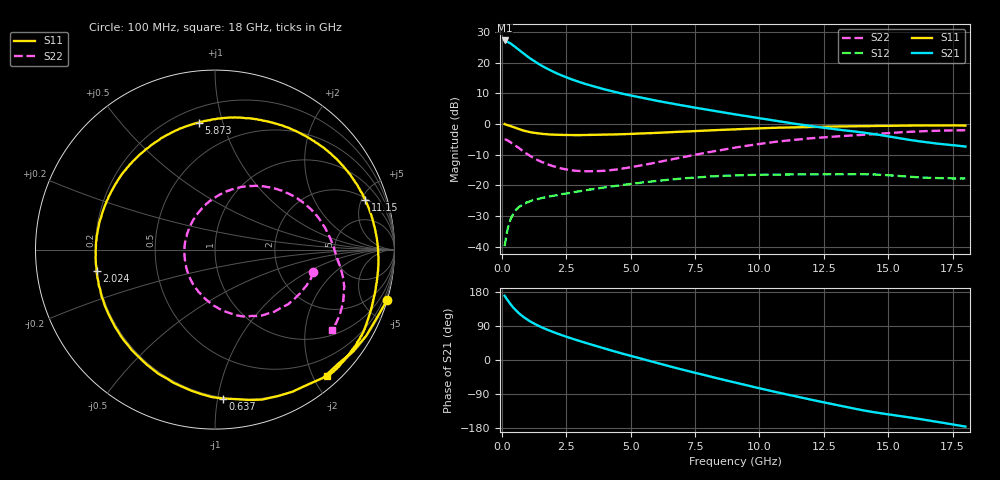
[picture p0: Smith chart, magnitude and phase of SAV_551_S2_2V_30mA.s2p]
! Data provided by Modelithics, Inc.  Tampa, Florida USA, June 2008
!Model SAV-551+
!VAR V_out= 2
!VAR I_out= 30
!VAR V_in= 0.3940
!VAR I_in= 0.9720
!BEGIN ACDATA
# GHZ S MA R 50
! Scattering Parameters
!% F n11x n11y n21x n21y n12x n12y n22x n22y
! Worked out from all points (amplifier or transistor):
!   401 points, 100 MHz to 18 GHz, reference 50 ohm
!   highest |S21| = 27.2 dB at 100 MHz (marker M1)
!   |S21| within 3 dB of that: start of sweep to 648.8 MHz
!   unconditionally stable (mu >= 1): 4.174 GHz to 10.93 GHz
!   at 3.054 GHz: K = 0.88, MSG = 17.7 dB, |S12| = -21.8 dB
!   at 9.05 GHz: K = 1.05, MAG = 8.5 dB, |S12| = -16.7 dB
!   at 18 GHz: K = 0.92, MSG = 5.2 dB, |S12| = -17.7 dB
!   lowest NFmin = 0.10 dB at 500 MHz
!   S11 on the Smith chart (normalised r, x): 100 MHz: 0.02, -6.95; 637 MHz: 0.19, -1.04; 2.024 GHz: 0.20, -0.09; 5.873 GHz: 0.29, +0.84; 11.15 GHz: 2.13, +5.34; 18 GHz: 0.17, -2.21
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0.1  0.9992 -16.4  22.85 169.8  0.01031 79.9  0.558 -12.7
0.1895  0.9698 -29.6  21.86 160.5  0.01708 74.1  0.547 -21.7
0.279  0.9361 -42.6  20.92 151.7  0.02351 68.3  0.5207 -31.8
0.3685  0.9117 -55.8  19.9 143.8  0.03038 61.0  0.4905 -41.4
0.50275  0.8757 -72.6  18.12 133.4  0.03843 54.9  0.4515 -54.4
0.637  0.8314 -86.9  16.32 124.5  0.04429 48.5  0.4138 -64.9
0.77125  0.7974 -99.4  14.71 116.9  0.0483 43.3  0.3734 -74.4
0.9055  0.7665 -110.5  13.31 110.1  0.05123 39.5  0.34 -82.9
1.174  0.727 -129.6  11.06 98.8  0.05726 33.5  0.2883 -98.2
1.532  0.6932 -149.1  8.916 86.5  0.0626 28.6  0.2417 -115.5
2.02425  0.6706 -169.8  6.978 72.8  0.06854 23.6  0.2038 -136.1
2.56125  0.662 172.3  5.611 59.9  0.07516 19.4  0.1805 -156.3
3.09825  0.6598 157.0  4.674 48.3  0.08178 15.0  0.171 -174.6
4.396  0.6761 126.3  3.312 22.2  0.09845 5.0  0.1811 146.3
5.87275  0.7135 97.1  2.449 -5.3  0.1169 -8.9  0.2305 111.6
6.0965  0.7216 93.2  2.353 -9.3  0.1197 -11.3  0.2418 107.4
7.439  0.7649 70.8  1.862 -32.8  0.134 -25.6  0.3126 83.6
9.05  0.8181 46.9  1.435 -59.3  0.1462 -43.6  0.4126 59.2
11.15325  0.8819 18.4  1.043 -92.3  0.1512 -67.8  0.5425 31.2
12.04825  0.8983 7.5  0.9212 -105.3  0.1517 -77.7  0.5887 20.5
15.0465  0.9348 -23.6  0.6259 -143.9  0.1466 -107.9  0.7125 -9.4
18  0.9427 -48.5  0.4307 -175.7  0.1298 -132.5  0.7914 -34.3
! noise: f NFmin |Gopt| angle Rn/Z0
0.5  0.1  0.322  24.68  0.069
0.7  0.139  0.3318  36.52  0.061
0.9  0.179  0.3413  48.1  0.055
1  0.198  0.346  53.79  0.052
1.9  0.375  0.3855  102.1  0.034
2.4  0.474  0.4054  126.7  0.031
3  0.591  0.4273  154.1  0.034
3.9  0.768  0.4563  -169.3  0.053
5  0.984  0.4853  -131.5  0.098
6  1.181  0.5055  -104  0.161
